(* Logix 5000 AddOnInstructionDefinition export Banner_Q76_Param_v4; software revision 33.00 *)

TYPE Banner_IOL_Port_v4 :   // UDT that has all of the data items necessary to communicate with a specific Port on a IO-Link Master
STRUCT
   Port_Controlled : INT;   // Each bit represents a port on an IO-Link Master. Set to 1 to tell AOI to control that port.
   Port_Activate : INT;   // Each bit represents a port on an IO-Link Master. When ON that port will process any commands in queue.
   Port_Read : INT;   // Each bit represents a port on an IO-Link Master. Used to determine when device AOI has requested a Read command.
   Port_Write : INT;   // Each bit represents a port on an IO-Link Master. Used to determine when device AOI has requested a Write command.
   Port_RW_Complete : INT;   // Each bit represents a port on an IO-Link Master. Tells device AOI that Read or Write request has been completed.
   Port_Device_Read : INT;
   Data_Transfer : SINT[190];   // Array to transfer data from IO-Master to device AOIs.
END_STRUCT
END_TYPE

TYPE Banner_Q76_RD_v4 :   // All of the read parameters for a Q76.
STRUCT
   Master_Cycle_Time : INT;
   Min_Cycle_Time : INT;
   M_Sequence_Capability : INT;
   IO_Link_Version_ID : INT;
   Process_Data_Input_Length : INT;
   Process_Data_Output_Length : INT;
   Combined_Vendor_ID : DINT;   // IO-Link Vendor ID
   Vendor_ID1 : INT;
   Vendor_ID2 : INT;
   Combined_Device_ID : DINT;   // IO-Link Device ID
   Device_ID1 : INT;
   Device_ID2 : INT;
   Device_ID3 : INT;
   PDI_Content : SINT;   // 0 = Switching Signal and Status, 1 = Analog ADC value and Switching Signal
   Status_Teach_or_Command : SINT;   // 0 = Finished, 1 = Running
   Command_Accepted : SINT;   // 0 = No, 1 = Yes
   Teach_Error : SINT;   // 0 = No, 1 = Yes
   Last_Values_Restored : SINT;   // 0 = No, 1 = Yes
   Reception_Level_too_High : SINT;   // 0 = No, 1 = Yes
   Reception_Level_too_Low : SINT;   // 0 = No, 1 = Yes
END_STRUCT
END_TYPE

TYPE Banner_Q76_v4 :   // All of the parameters for a Q76.
STRUCT
   Initial_Global_Read : BOOL;   // Determines if all of the IO-Link data has been read into the PLC yet
   Command : INT;   // Value placed in here will activate a read or write to a specifc IO-Link Index
   Read_Data : Banner_Q76_RD_v4;   // Read Only Data
   Write_Data : Banner_Q76_WD_v4;   // Write Data
   Archive : Banner_Q76_WD_v4;   // Archive Data
   Reset : BOOL;   // Resets AOI. This will force a complete parameter read of the sensor.
END_STRUCT
END_TYPE

TYPE Banner_Q76_WD_v4 :   // UDT that stores the Write Data for a S15C.
STRUCT
   Standard_Command : INT;   // See IODD file for list of commands that can be activated via the System Command interface
   Off_Limit : INT;
   On_Limit : INT;
   Key_Lock : SINT;   // 0 = Disabled, 1 = Enabled
   Q2_Logic_Function : SINT;   // 0 = Inverted Switching Output, 1 = Switching Output, 2 = Warning Output
   Delay_Function : SINT;   // 0 = On Delay, 1 = Off Delay, 2 = Pulse Stretching, 3 = Pulse Suppression
   Timer_Base : SINT;   // 0 = 1ms, 1 = 10ms, 2 = 100ms, 3 = 1000ms
   Multiplication_Factor : SINT;   // 1 to 15
   Easy_Tune : SINT;   // 0 = Disabled, 1 = Enabled
   Light_Dark_Switching : SINT;   // 0 = light, 1 = dark
   Internal_Delay_Unit : SINT;   // 0 = Disabled, 1 = Enabled
   Teach_Value_2 : INT;
END_STRUCT
END_TYPE

ADD_ON_INSTRUCTION Banner_Q76_Param_v4   (* revision 4.0, vendor Banner Engineering *)
// AOI to read and write parameter data to an IO-Link Q76.
VAR_IN_OUT
   Q76 : Banner_Q76_v4; {required}
   Port_Data : Banner_IOL_Port_v4; {required}
END_VAR
VAR_INPUT
   Port : DINT; {required}
END_VAR
VAR
   Local_Control : DINT; {access None}
   Global_Read_Command_Value : INT; {access None}
   Global_Write_Command_Value : INT; {access None}
   Error_Generated : BOOL; {access None}
   Command_Being_Processed : BOOL; {access None}
   Index_Write_Inprocess : INT; {access None}
   Index_Write_Control : INT; {access None}
   Update_Archive : BOOL; {access None}
   Inprocess_Index : DINT; {access None}
END_VAR

ROUTINE Logic   (* ladder *)
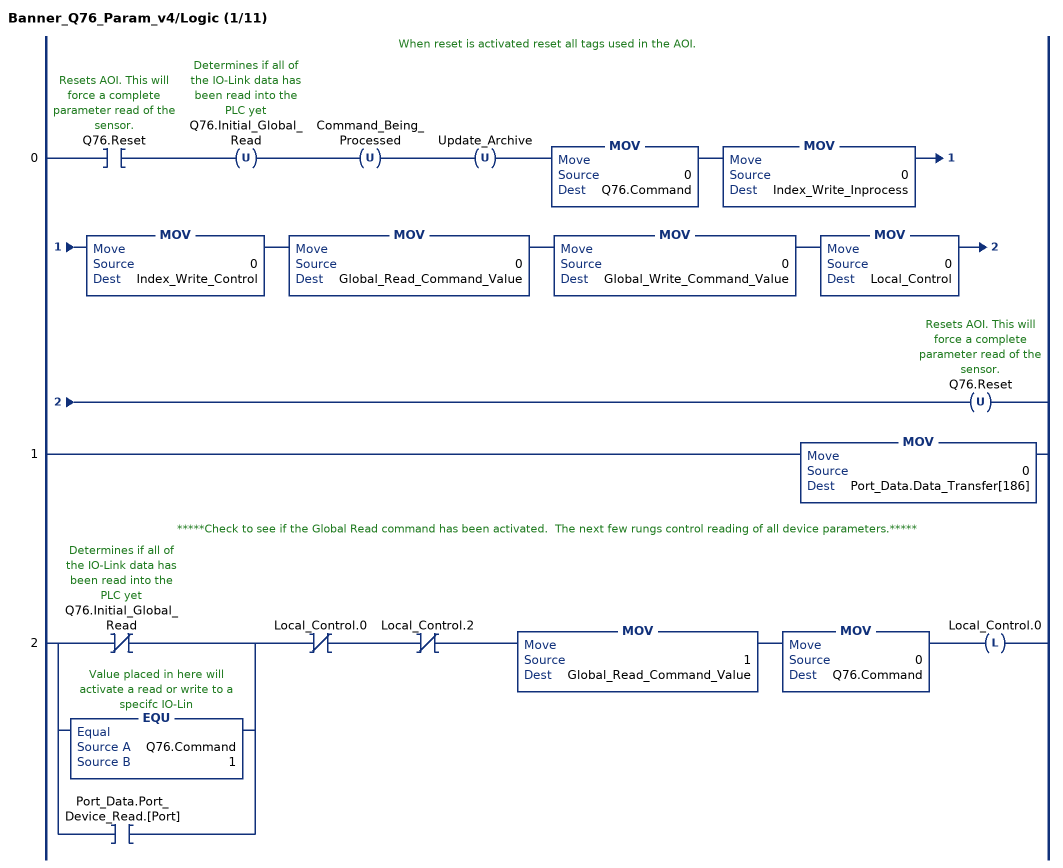
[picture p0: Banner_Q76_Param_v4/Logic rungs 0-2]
   // When reset is activated reset all tags used in the AOI.
   0: XIC(Q76.Reset)OTU(Q76.Initial_Global_Read)OTU(Command_Being_Processed)OTU(Update_Archive)MOV(0,Q76.Command)MOV(0,Index_Write_Inprocess)MOV(0,Index_Write_Control)MOV(0,Global_Read_Command_Value)MOV(0,Global_Write_Command_Value)MOV(0,Local_Control)OTU(Q76.Reset);
   1: MOV(0,Port_Data.Data_Transfer[186]);
   // *****Check to see if the Global Read command has been activated.  The next few rungs control reading of all device parameters.*****
   2: [XIO(Q76.Initial_Global_Read) ,EQU(Q76.Command,1) ,XIC(Port_Data.Port_Device_Read.[Port]) ]XIO(Local_Control.0)XIO(Local_Control.2)MOV(1,Global_Read_Command_Value)MOV(0,Q76.Command)OTL(Local_Control.0);
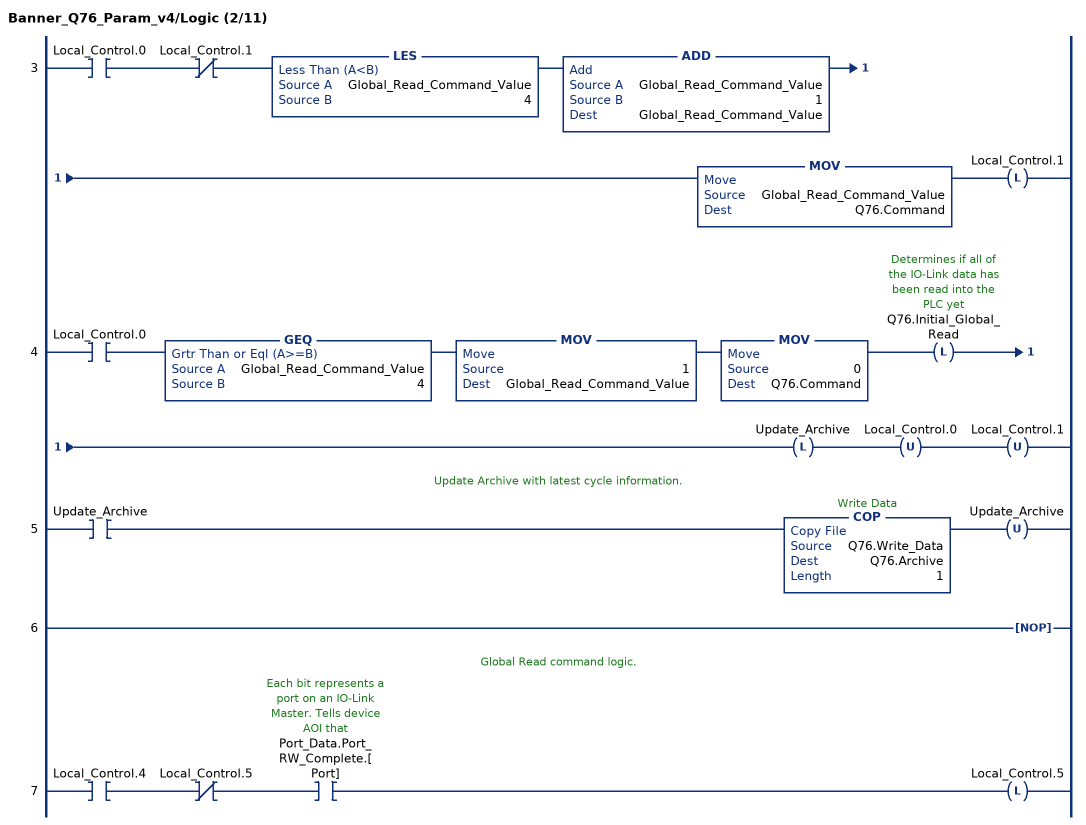
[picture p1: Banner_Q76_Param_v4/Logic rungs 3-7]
   3: XIC(Local_Control.0)XIO(Local_Control.1)LES(Global_Read_Command_Value,4)ADD(Global_Read_Command_Value,1,Global_Read_Command_Value)MOV(Global_Read_Command_Value,Q76.Command)OTL(Local_Control.1);
   4: XIC(Local_Control.0)GEQ(Global_Read_Command_Value,4)MOV(1,Global_Read_Command_Value)MOV(0,Q76.Command)OTL(Q76.Initial_Global_Read)OTL(Update_Archive)OTU(Local_Control.0)OTU(Local_Control.1);
   // Update Archive with latest cycle information.
   5: XIC(Update_Archive)COP(Q76.Write_Data,Q76.Archive,1)OTU(Update_Archive);
   6: NOP();
   // Global Read command logic.
   7: XIC(Local_Control.4)XIO(Local_Control.5)XIC(Port_Data.Port_RW_Complete.[Port])OTL(Local_Control.5);
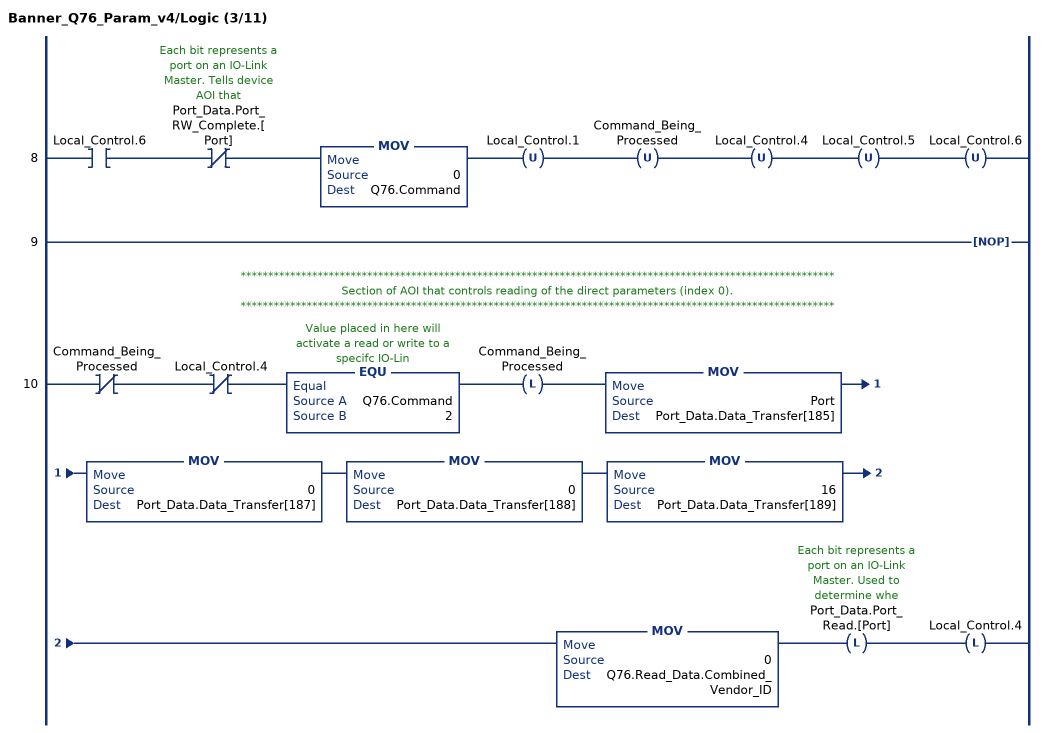
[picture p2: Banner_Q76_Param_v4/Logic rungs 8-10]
   8: XIC(Local_Control.6)XIO(Port_Data.Port_RW_Complete.[Port])MOV(0,Q76.Command)OTU(Local_Control.1)OTU(Command_Being_Processed)OTU(Local_Control.4)OTU(Local_Control.5)OTU(Local_Control.6);
   9: NOP();
   // ************************************************************************************************************
   // Section of AOI that controls reading of the direct parameters (index 0).
   // ************************************************************************************************************
   10: XIO(Command_Being_Processed)XIO(Local_Control.4)EQU(Q76.Command,2)OTL(Command_Being_Processed)MOV(Port,Port_Data.Data_Transfer[185])MOV(0,Port_Data.Data_Transfer[187])MOV(0,Port_Data.Data_Transfer[188])MOV(16,Port_Data.Data_Transfer[189])MOV(0,Q76.Read_Data.Combined_Vendor_ID)OTL(Port_Data.Port_Read.[Port])OTL(Local_Control.4);
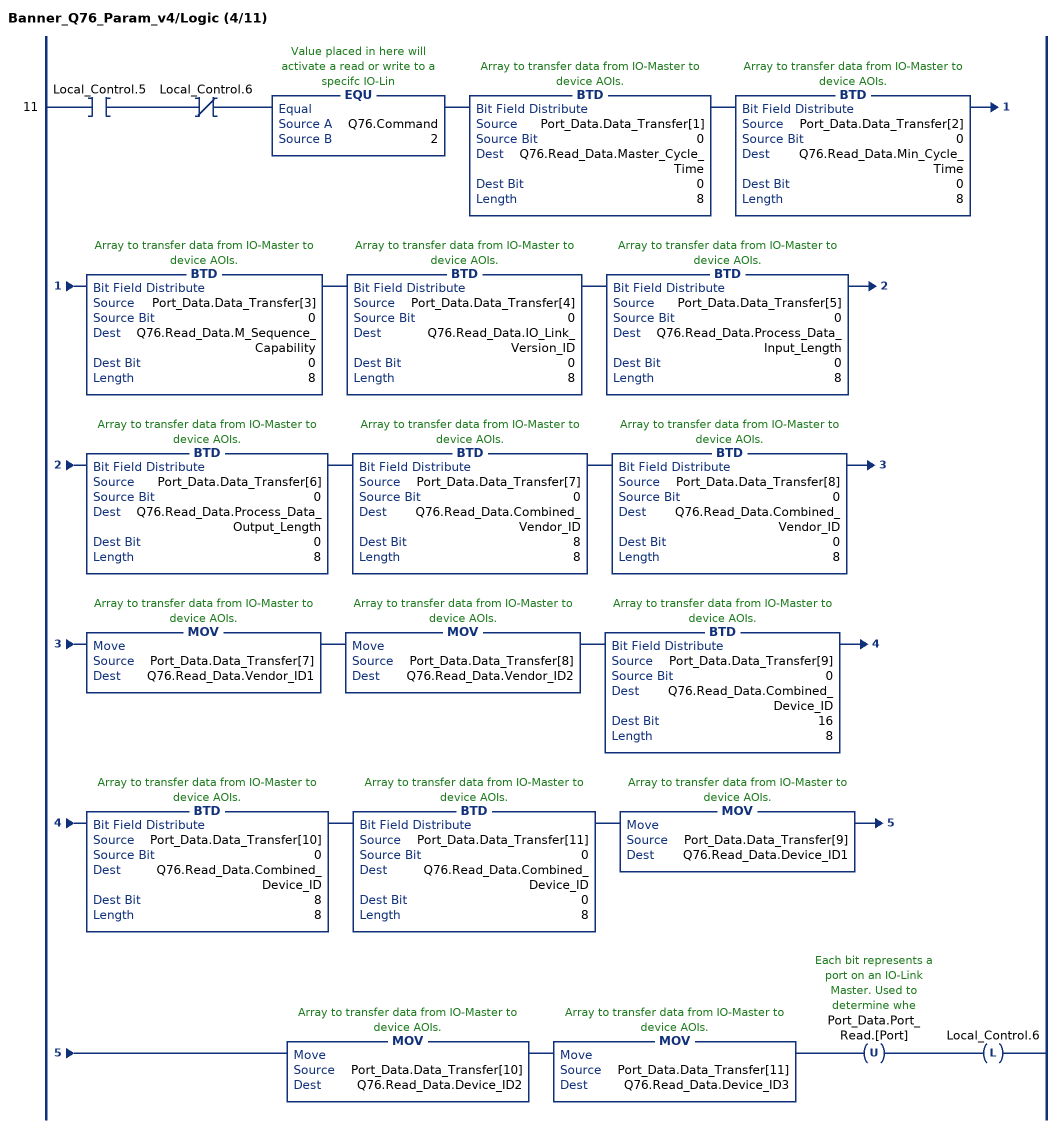
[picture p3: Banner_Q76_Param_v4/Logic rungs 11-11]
   11: XIC(Local_Control.5)XIO(Local_Control.6)EQU(Q76.Command,2)BTD(Port_Data.Data_Transfer[1],0,Q76.Read_Data.Master_Cycle_Time,0,8)BTD(Port_Data.Data_Transfer[2],0,Q76.Read_Data.Min_Cycle_Time,0,8)BTD(Port_Data.Data_Transfer[3],0,Q76.Read_Data.M_Sequence_Capability,0,8)BTD(Port_Data.Data_Transfer[4],0,Q76.Read_Data.IO_Link_Version_ID,0,8)BTD(Port_Data.Data_Transfer[5],0,Q76.Read_Data.Process_Data_Input_Length,0,8)BTD(Port_Data.Data_Transfer[6],0,Q76.Read_Data.Process_Data_Output_Length,0,8)BTD(Port_Data.Data_Transfer[7],0,Q76.Read_Data.Combined_Vendor_ID,8,8)BTD(Port_Data.Data_Transfer[8],0,Q76.Read_Data.Combined_Vendor_ID,0,8)MOV(Port_Data.Data_Transfer[7],Q76.Read_Data.Vendor_ID1)MOV(Port_Data.Data_Transfer[8],Q76.Read_Data.Vendor_ID2)BTD(Port_Data.Data_Transfer[9],0,Q76.Read_Data.Combined_Device_ID,16,8)BTD(Port_Data.Data_Transfer[10],0,Q76.Read_Data.Combined_Device_ID,8,8)BTD(Port_Data.Data_Transfer[11],0,Q76.Read_Data.Combined_Device_ID,0,8)MOV(Port_Data.Data_Transfer[9],Q76.Read_Data.Device_ID1)MOV(Port_Data.Data_Transfer[10],Q76.Read_Data.Device_ID2)MOV(Port_Data.Data_Transfer[11],Q76.Read_Data.Device_ID3)OTU(Port_Data.Port_Read.[Port])OTL(Local_Control.6);
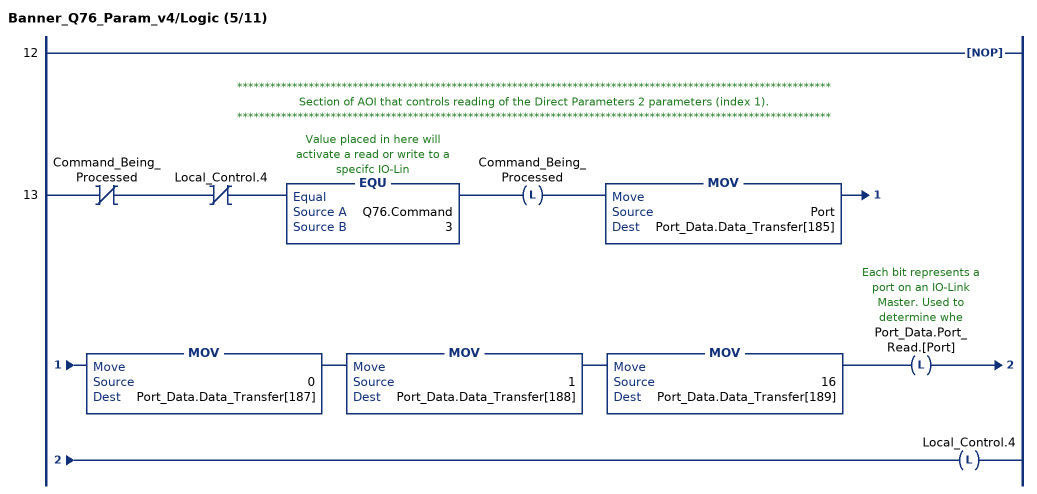
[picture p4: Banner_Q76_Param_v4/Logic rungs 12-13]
   12: NOP();
   // ************************************************************************************************************
   // Section of AOI that controls reading of the Direct Parameters 2 parameters (index 1).
   // ************************************************************************************************************
   13: XIO(Command_Being_Processed)XIO(Local_Control.4)EQU(Q76.Command,3)OTL(Command_Being_Processed)MOV(Port,Port_Data.Data_Transfer[185])MOV(0,Port_Data.Data_Transfer[187])MOV(1,Port_Data.Data_Transfer[188])MOV(16,Port_Data.Data_Transfer[189])OTL(Port_Data.Port_Read.[Port])OTL(Local_Control.4);
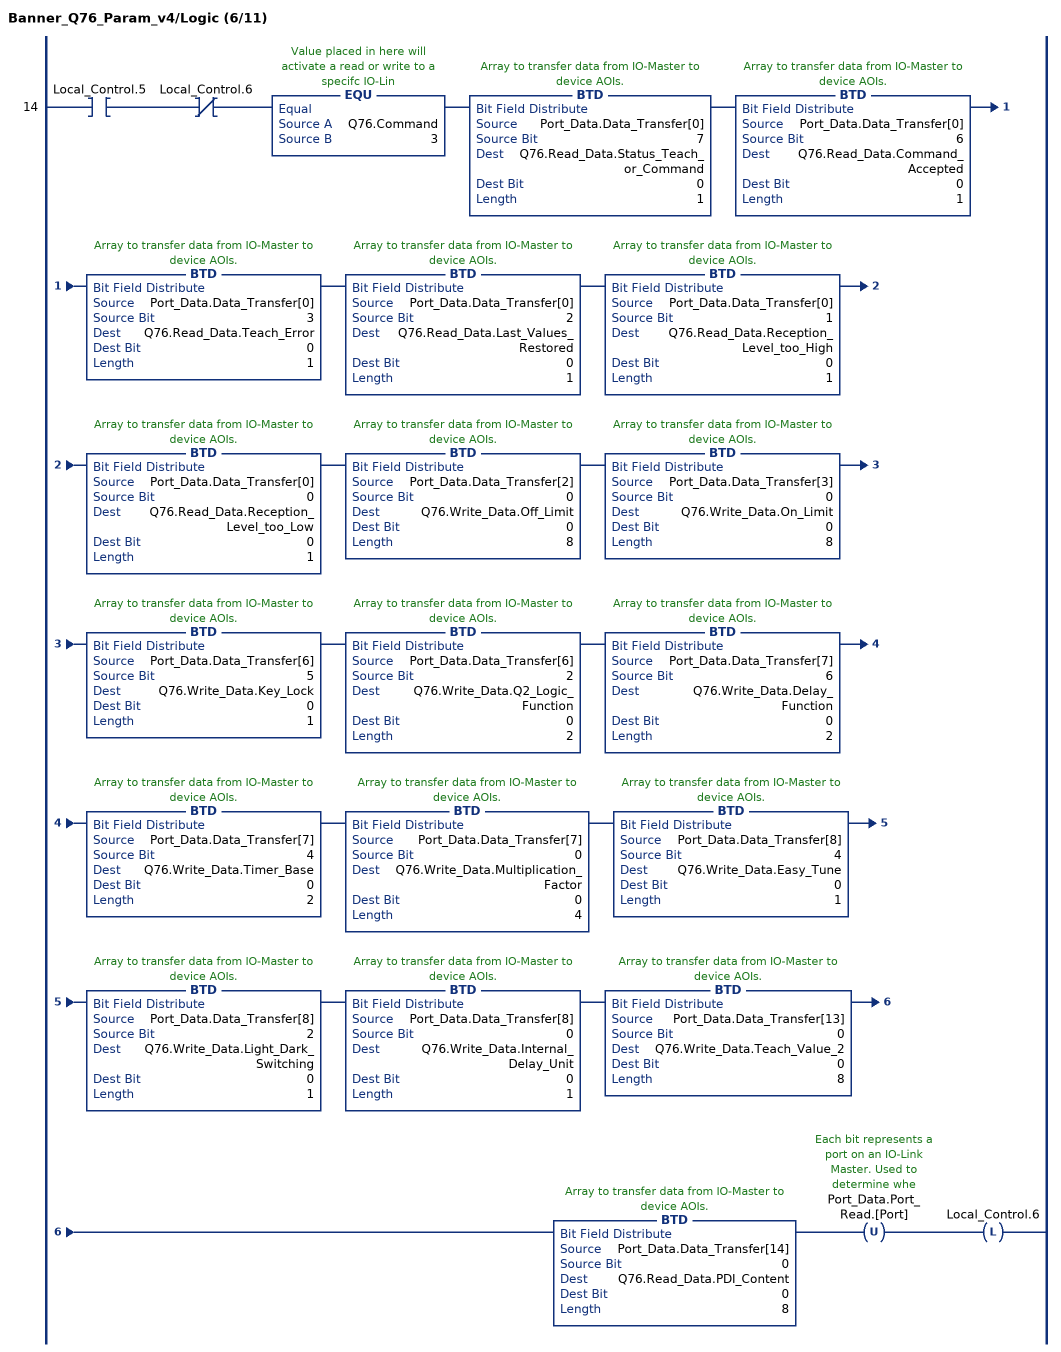
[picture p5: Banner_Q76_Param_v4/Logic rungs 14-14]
   14: XIC(Local_Control.5)XIO(Local_Control.6)EQU(Q76.Command,3)BTD(Port_Data.Data_Transfer[0],7,Q76.Read_Data.Status_Teach_or_Command,0,1)BTD(Port_Data.Data_Transfer[0],6,Q76.Read_Data.Command_Accepted,0,1)BTD(Port_Data.Data_Transfer[0],3,Q76.Read_Data.Teach_Error,0,1)BTD(Port_Data.Data_Transfer[0],2,Q76.Read_Data.Last_Values_Restored,0,1)BTD(Port_Data.Data_Transfer[0],1,Q76.Read_Data.Reception_Level_too_High,0,1)BTD(Port_Data.Data_Transfer[0],0,Q76.Read_Data.Reception_Level_too_Low,0,1)BTD(Port_Data.Data_Transfer[2],0,Q76.Write_Data.Off_Limit,0,8)BTD(Port_Data.Data_Transfer[3],0,Q76.Write_Data.On_Limit,0,8)BTD(Port_Data.Data_Transfer[6],5,Q76.Write_Data.Key_Lock,0,1)BTD(Port_Data.Data_Transfer[6],2,Q76.Write_Data.Q2_Logic_Function,0,2)BTD(Port_Data.Data_Transfer[7],6,Q76.Write_Data.Delay_Function,0,2)BTD(Port_Data.Data_Transfer[7],4,Q76.Write_Data.Timer_Base,0,2)BTD(Port_Data.Data_Transfer[7],0,Q76.Write_Data.Multiplication_Factor,0,4)BTD(Port_Data.Data_Transfer[8],4,Q76.Write_Data.Easy_Tune,0,1)BTD(Port_Data.Data_Transfer[8],2,Q76.Write_Data.Light_Dark_Switching,0,1)BTD(Port_Data.Data_Transfer[8],0,Q76.Write_Data.Internal_Delay_Unit,0,1)BTD(Port_Data.Data_Transfer[13],0,Q76.Write_Data.Teach_Value_2,0,8)BTD(Port_Data.Data_Transfer[14],0,Q76.Read_Data.PDI_Content,0,8)OTU(Port_Data.Port_Read.[Port])OTL(Local_Control.6);
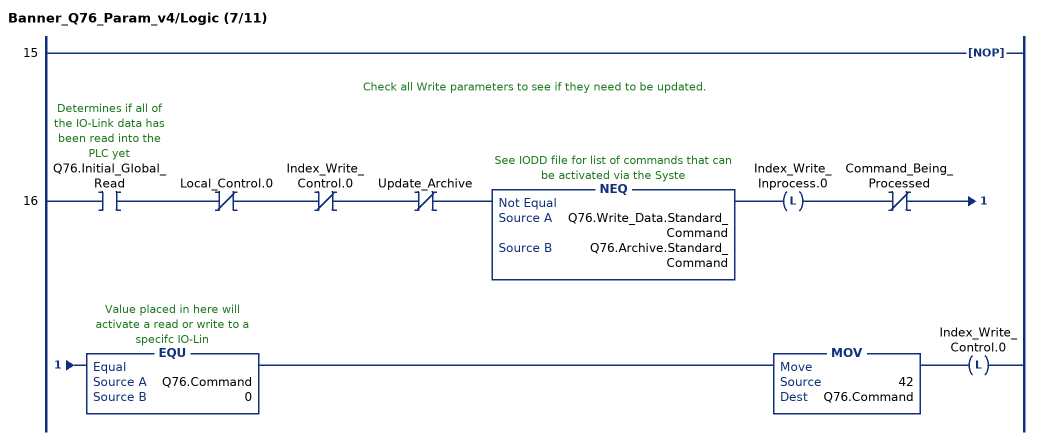
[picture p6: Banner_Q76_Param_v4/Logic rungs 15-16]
   15: NOP();
   // Check all Write parameters to see if they need to be updated.
   16: XIC(Q76.Initial_Global_Read)XIO(Local_Control.0)XIO(Index_Write_Control.0)XIO(Update_Archive)NEQ(Q76.Write_Data.Standard_Command,Q76.Archive.Standard_Command)OTL(Index_Write_Inprocess.0)XIO(Command_Being_Processed)EQU(Q76.Command,0)MOV(42,Q76.Command)OTL(Index_Write_Control.0);
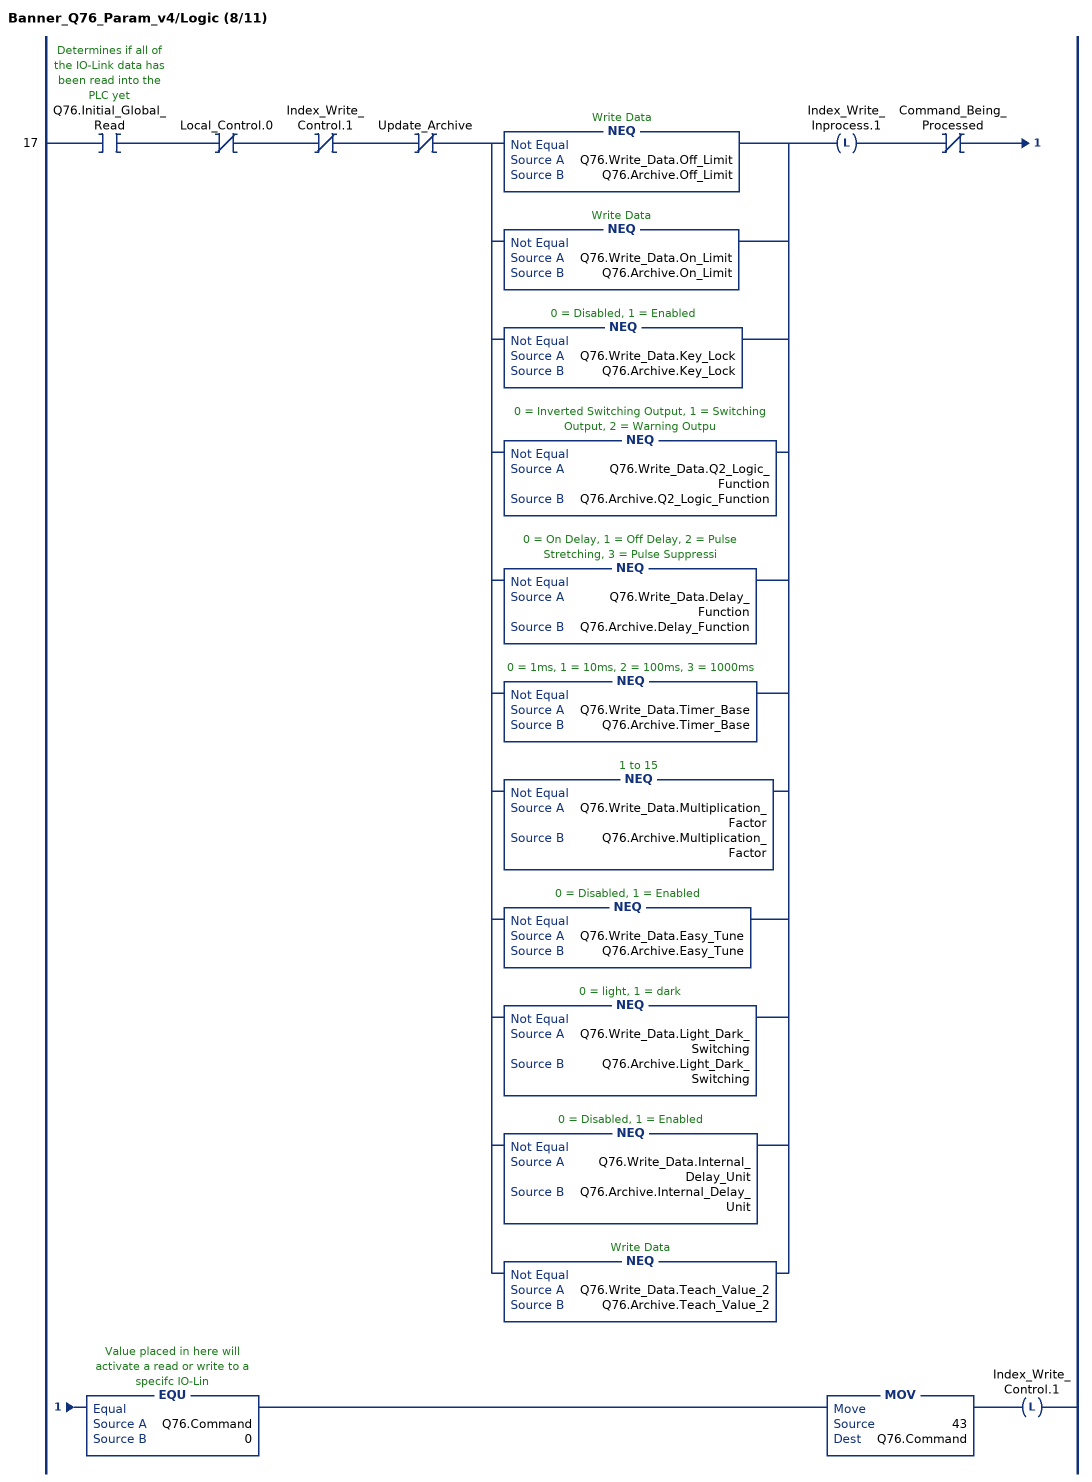
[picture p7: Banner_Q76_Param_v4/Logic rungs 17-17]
   17: XIC(Q76.Initial_Global_Read)XIO(Local_Control.0)XIO(Index_Write_Control.1)XIO(Update_Archive)[NEQ(Q76.Write_Data.Off_Limit,Q76.Archive.Off_Limit) ,NEQ(Q76.Write_Data.On_Limit,Q76.Archive.On_Limit) ,NEQ(Q76.Write_Data.Key_Lock,Q76.Archive.Key_Lock) ,NEQ(Q76.Write_Data.Q2_Logic_Function,Q76.Archive.Q2_Logic_Function) ,NEQ(Q76.Write_Data.Delay_Function,Q76.Archive.Delay_Function) ,NEQ(Q76.Write_Data.Timer_Base,Q76.Archive.Timer_Base) ,NEQ(Q76.Write_Data.Multiplication_Factor,Q76.Archive.Multiplication_Factor) ,NEQ(Q76.Write_Data.Easy_Tune,Q76.Archive.Easy_Tune) ,NEQ(Q76.Write_Data.Light_Dark_Switching,Q76.Archive.Light_Dark_Switching) ,NEQ(Q76.Write_Data.Internal_Delay_Unit,Q76.Archive.Internal_Delay_Unit) ,NEQ(Q76.Write_Data.Teach_Value_2,Q76.Archive.Teach_Value_2) ]OTL(Index_Write_Inprocess.1)XIO(Command_Being_Processed)EQU(Q76.Command,0)MOV(43,Q76.Command)OTL(Index_Write_Control.1);
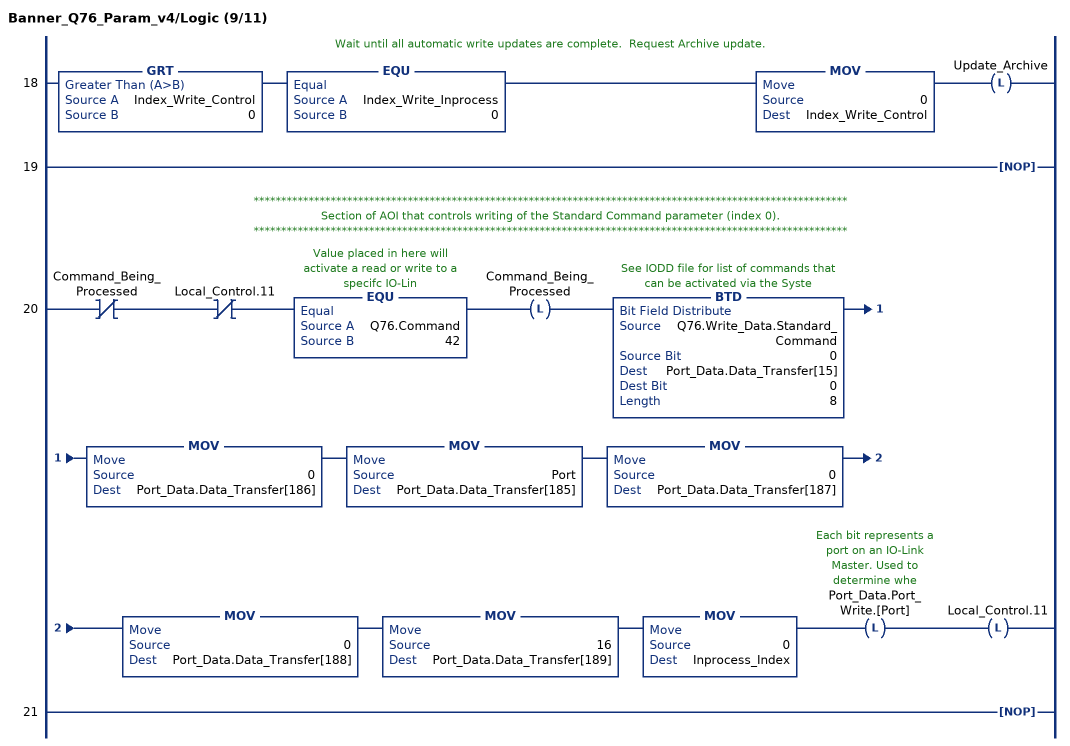
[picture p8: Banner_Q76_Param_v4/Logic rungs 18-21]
   // Wait until all automatic write updates are complete.  Request Archive update.
   18: GRT(Index_Write_Control,0)EQU(Index_Write_Inprocess,0)MOV(0,Index_Write_Control)OTL(Update_Archive);
   19: NOP();
   // ************************************************************************************************************
   // Section of AOI that controls writing of the Standard Command parameter (index 0).
   // ************************************************************************************************************
   20: XIO(Command_Being_Processed)XIO(Local_Control.11)EQU(Q76.Command,42)OTL(Command_Being_Processed)BTD(Q76.Write_Data.Standard_Command,0,Port_Data.Data_Transfer[15],0,8)MOV(0,Port_Data.Data_Transfer[186])MOV(Port,Port_Data.Data_Transfer[185])MOV(0,Port_Data.Data_Transfer[187])MOV(0,Port_Data.Data_Transfer[188])MOV(16,Port_Data.Data_Transfer[189])MOV(0,Inprocess_Index)OTL(Port_Data.Port_Write.[Port])OTL(Local_Control.11);
   21: NOP();
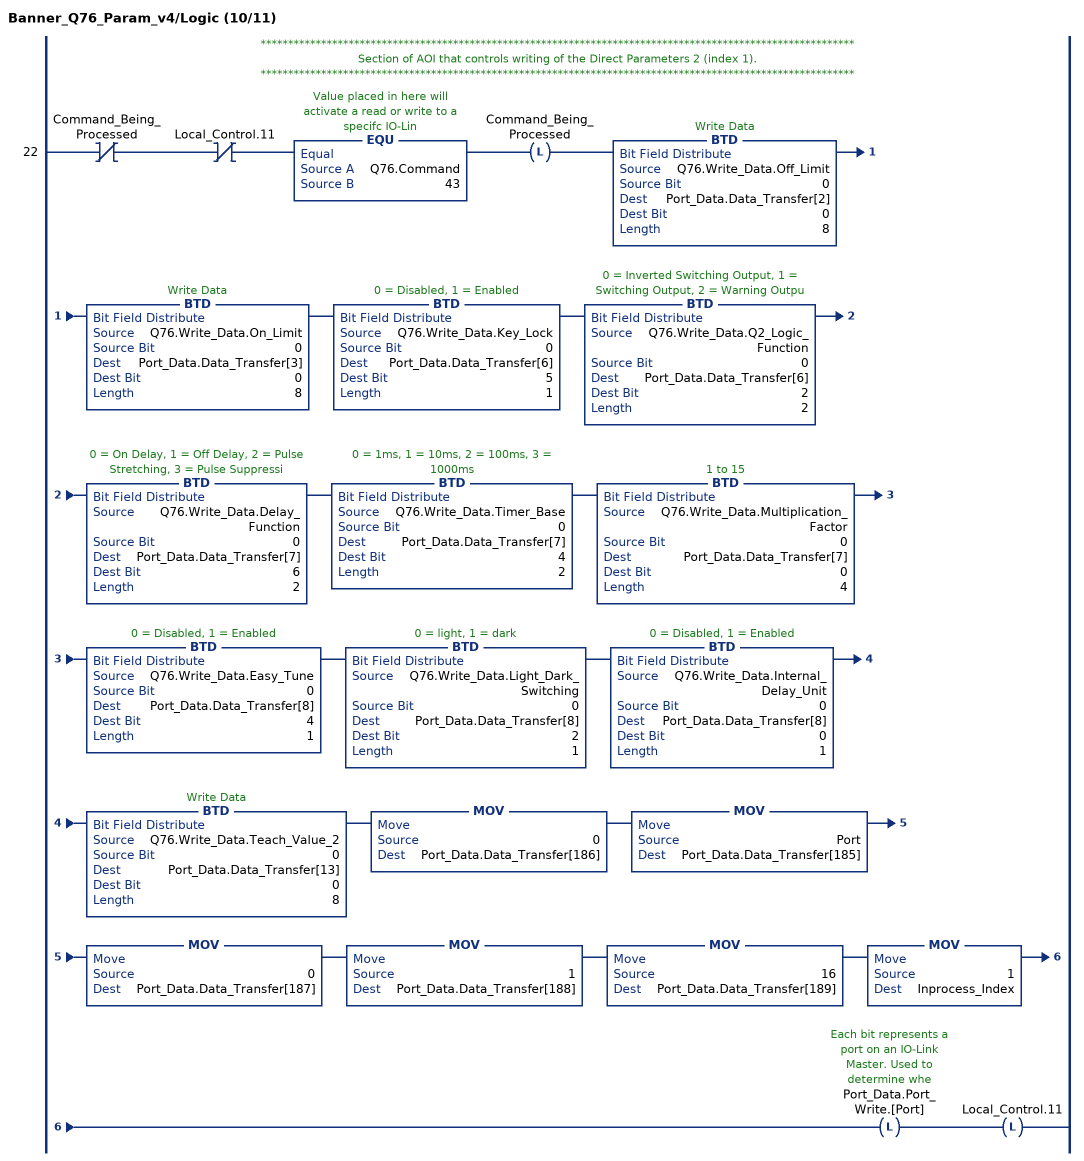
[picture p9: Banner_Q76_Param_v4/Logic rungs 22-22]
   // ************************************************************************************************************
   // Section of AOI that controls writing of the Direct Parameters 2 (index 1).
   // ************************************************************************************************************
   22: XIO(Command_Being_Processed)XIO(Local_Control.11)EQU(Q76.Command,43)OTL(Command_Being_Processed)BTD(Q76.Write_Data.Off_Limit,0,Port_Data.Data_Transfer[2],0,8)BTD(Q76.Write_Data.On_Limit,0,Port_Data.Data_Transfer[3],0,8)BTD(Q76.Write_Data.Key_Lock,0,Port_Data.Data_Transfer[6],5,1)BTD(Q76.Write_Data.Q2_Logic_Function,0,Port_Data.Data_Transfer[6],2,2)BTD(Q76.Write_Data.Delay_Function,0,Port_Data.Data_Transfer[7],6,2)BTD(Q76.Write_Data.Timer_Base,0,Port_Data.Data_Transfer[7],4,2)BTD(Q76.Write_Data.Multiplication_Factor,0,Port_Data.Data_Transfer[7],0,4)BTD(Q76.Write_Data.Easy_Tune,0,Port_Data.Data_Transfer[8],4,1)BTD(Q76.Write_Data.Light_Dark_Switching,0,Port_Data.Data_Transfer[8],2,1)BTD(Q76.Write_Data.Internal_Delay_Unit,0,Port_Data.Data_Transfer[8],0,1)BTD(Q76.Write_Data.Teach_Value_2,0,Port_Data.Data_Transfer[13],0,8)MOV(0,Port_Data.Data_Transfer[186])MOV(Port,Port_Data.Data_Transfer[185])MOV(0,Port_Data.Data_Transfer[187])MOV(1,Port_Data.Data_Transfer[188])MOV(16,Port_Data.Data_Transfer[189])MOV(1,Inprocess_Index)OTL(Port_Data.Port_Write.[Port])OTL(Local_Control.11);
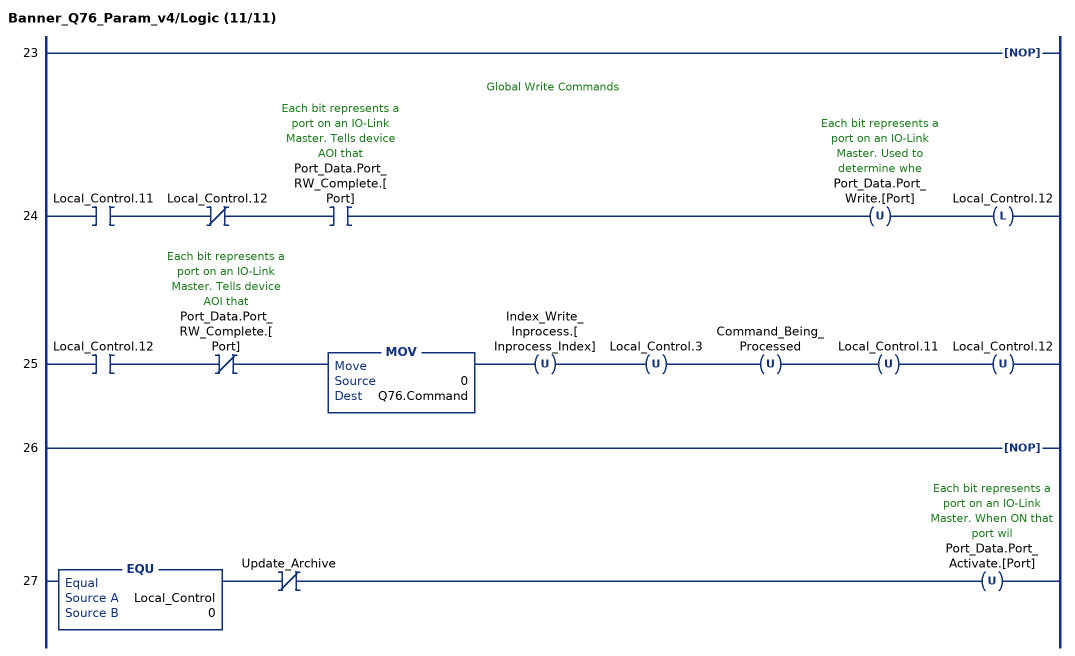
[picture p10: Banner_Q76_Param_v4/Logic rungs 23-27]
   23: NOP();
   // Global Write Commands
   24: XIC(Local_Control.11)XIO(Local_Control.12)XIC(Port_Data.Port_RW_Complete.[Port])OTU(Port_Data.Port_Write.[Port])OTL(Local_Control.12);
   25: XIC(Local_Control.12)XIO(Port_Data.Port_RW_Complete.[Port])MOV(0,Q76.Command)OTU(Index_Write_Inprocess.[Inprocess_Index])OTU(Local_Control.3)OTU(Command_Being_Processed)OTU(Local_Control.11)OTU(Local_Control.12);
   26: NOP();
   27: EQU(Local_Control,0)XIO(Update_Archive)OTU(Port_Data.Port_Activate.[Port]);
END_ROUTINE
END_ADD_ON_INSTRUCTION
